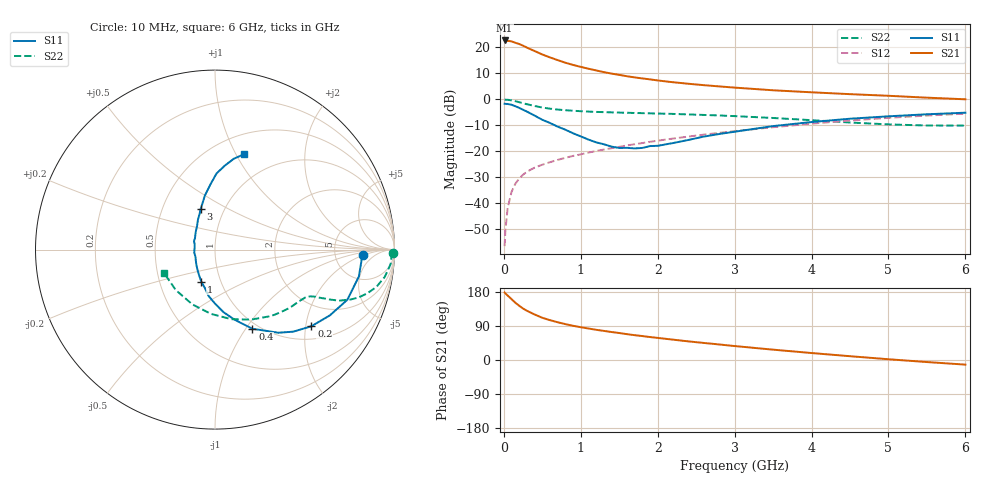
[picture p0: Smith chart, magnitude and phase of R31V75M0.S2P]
! SIEMENS Small Signal Semiconductors
! BFR181
! Si NPN RF Bipolar Junction Transistor in SOT23
! VCE = 1.75 V  IC = 5 mA
! Common Emitter S-Parameters:  May  1996
# GHz  S  MA  R  50
!  f  S11  S21  S12  S22
! GHz  MAG  ANG  MAG  ANG  MAG  ANG  MAG  ANG
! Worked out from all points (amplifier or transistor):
!   36 points, 10 MHz to 6 GHz, reference 50 ohm
!   highest |S21| = 22.7 dB at 10 MHz (marker M1)
!   |S21| within 3 dB of that: start of sweep to 318.7 MHz
!   unconditionally stable (mu >= 1): 1.034 GHz to 2.96 GHz
!   at 250 MHz: K = 0.43, MSG = 24.8 dB, |S12| = -29.0 dB
!   at 1.4 GHz: K = 1.06, MAG = 12.8 dB, |S12| = -18.8 dB
!   at 6 GHz: K = 0.86, MSG = 2.8 dB, |S12| = -5.5 dB
!   S11 on the Smith chart (normalised r, x): 10 MHz: 10, -2; 200 MHz: 1.33, -2.15; 400 MHz: 0.93, -1.07; 1 GHz: 0.81, -0.30; 3 GHz: 0.77, +0.37; 6 GHz: 0.70, +1.08
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0.01  0.8255 -2.2  13.61 178.0  0.0015 90.3  0.9909 -1.0
0.02  0.8188 -4.1  13.33 175.8  0.003 85.7  0.9849 -1.9
0.05  0.8155 -10.6  13.4 170.0  0.0082 85.1  0.982 -4.7
0.1  0.7884 -20.8  13.05 160.6  0.0166 78.5  0.9583 -9.1
0.15  0.738 -29.7  12.27 151.0  0.0239 74.8  0.9232 -13.0
0.2  0.6862 -38.5  11.62 143.1  0.0301 71.5  0.8832 -16.0
0.25  0.6315 -46.4  10.79 135.7  0.0356 68.0  0.8437 -18.4
0.3  0.5822 -52.7  9.911 129.9  0.0406 66.3  0.8074 -20.1
0.4  0.4878 -64.7  8.514 120.1  0.0487 63.8  0.7467 -22.4
0.5  0.4053 -74.4  7.308 111.4  0.0554 62.8  0.6975 -23.5
0.6  0.3516 -82.3  6.417 105.1  0.0619 62.5  0.6624 -24.2
0.8  0.2609 -97.9  5.077 94.7  0.0753 62.4  0.6189 -25.1
1  0.1941 -113.2  4.216 86.5  0.0876 63.1  0.5922 -26.1
1.1  0.1685 -121.7  3.891 83.1  0.0948 63.6  0.5824 -26.7
1.3  0.1371 -138.4  3.346 76.8  0.1084 64.0  0.5681 -28.1
1.6  0.1169 -172.0  2.789 68.2  0.1299 63.9  0.5532 -31.0
2.2  0.1446 138.1  2.137 53.7  0.1764 62.4  0.5255 -38.4
3  0.2387 109.6  1.685 36.8  0.245 57.6  0.4766 -51.5
3.5  0.3063 100.6  1.497 27.3  0.2915 53.5  0.4389 -62.7
4.5  0.4247 88.8  1.261 10.0  0.392 43.1  0.3589 -93.5
5.5  0.517 78.3  1.079 -5.4  0.4886 30.2  0.3141 -134.0
6  0.5545 73.2  1.004 -12.2  0.532 23.0  0.3129 -155.9
